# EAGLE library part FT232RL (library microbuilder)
FTDI FT232RL USB TO RS232 Converter Digikey: 768-1007-1-ND
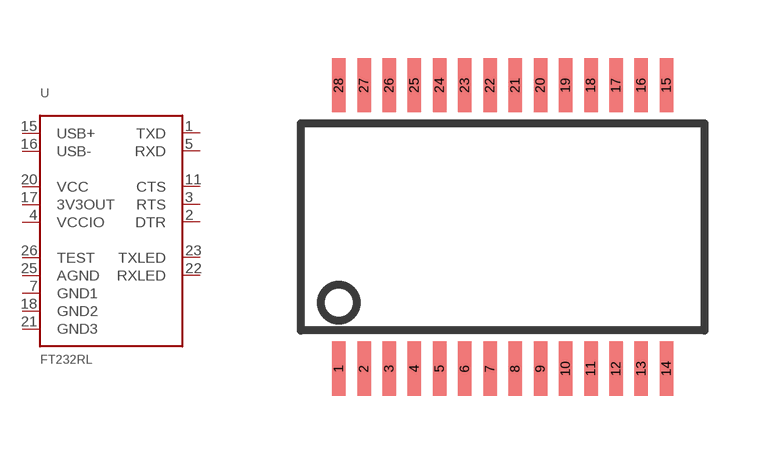
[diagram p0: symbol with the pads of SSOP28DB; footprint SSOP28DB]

Designator prefix U

## FT232RLSSOP28  [SSOP28DB]
1  TXD  out
2  DTR
3  RTS
4  VCCIO  pwr
5  RXD  in
7  GND1  pwr
11  CTS
15  USB+
16  USB-
17  3V3OUT  pwr
18  GND2  pwr
20  VCC  pwr
21  GND3  pwr
22  RXLED
23  TXLED
25  AGND  pwr
26  TEST  in

## Footprint SSOP28DB (pad centres in mm)
Small Shrink Outline Package
smd 0.348 x 1.397: 1 -4.225,-3.656; 2 -3.575,-3.656; 3 -2.925,-3.656; 4 -2.275,-3.656; 5 -1.625,-3.656; 6 -0.975,-3.656; 7 -0.325,-3.656; 8 0.325,-3.656; 9 0.975,-3.656; 10 1.625,-3.656; 11 2.275,-3.656; 12 2.925,-3.656; 13 3.575,-3.656; 14 4.225,-3.656; 15 4.225,3.656; 16 3.575,3.656; 17 2.925,3.656; 18 2.275,3.656; 19 1.625,3.656; 20 0.975,3.656; 21 0.325,3.656; 22 -0.325,3.656; 23 -0.975,3.656; 24 -1.625,3.656; 25 -2.275,3.656; 26 -2.925,3.656; 27 -3.575,3.656; 28 -4.225,3.656

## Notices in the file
This work is placed in the public domain, and may be freely used for commercial and non-commercial work with the following conditions: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
Shamelessly taken from the Adafruit Eagle library (public domain) ... thanks!
